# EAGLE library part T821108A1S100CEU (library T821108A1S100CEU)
HEADER, VERTICAL, 2.54MM, 8WAY Amphenol T821 Series, 2.54mm Pitch 8 Way 2 Row Straight PCB Header, Solder Termination, 3A Source: Datasheet
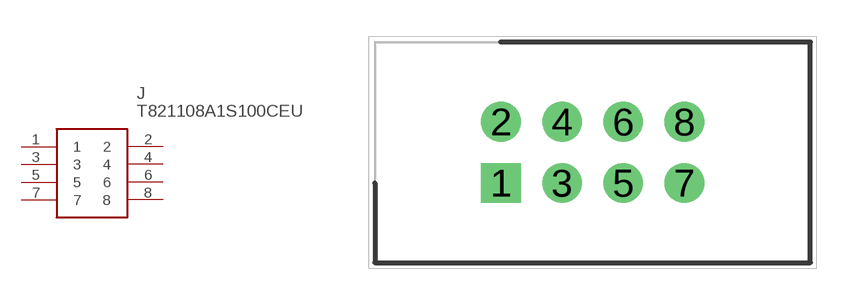
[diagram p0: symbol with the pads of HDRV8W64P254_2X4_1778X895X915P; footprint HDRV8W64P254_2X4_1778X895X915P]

Designator prefix J

## T821108A1S100CEU (Description: HEADER, VERTICAL, 2.54MM, 8WAY Amphenol T821 Series, 2.54mm Pitch 8 Way 2 Row Straight PCB Header, Solder Termination, 3A; Height: 9.15mm; Manufacturer_Name: Amphenol; Manufacturer_Part_Number: T821108A1S100CEU; RS_Part_Number: 1702738)  [HDRV8W64P254_2X4_1778X895X915P]
1  1
2  2
3  3
4  4
5  5
6  6
7  7
8  8

## Footprint HDRV8W64P254_2X4_1778X895X915P (pad centres in mm)
T821108A1S100CEU
drill 1.1 pad 1.65 square: 1 0,0
drill 1.1 pad 1.65: 2 0,2.54; 3 2.54,0; 4 2.54,2.54; 5 5.08,0; 6 5.08,2.54; 7 7.62,0; 8 7.62,2.54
